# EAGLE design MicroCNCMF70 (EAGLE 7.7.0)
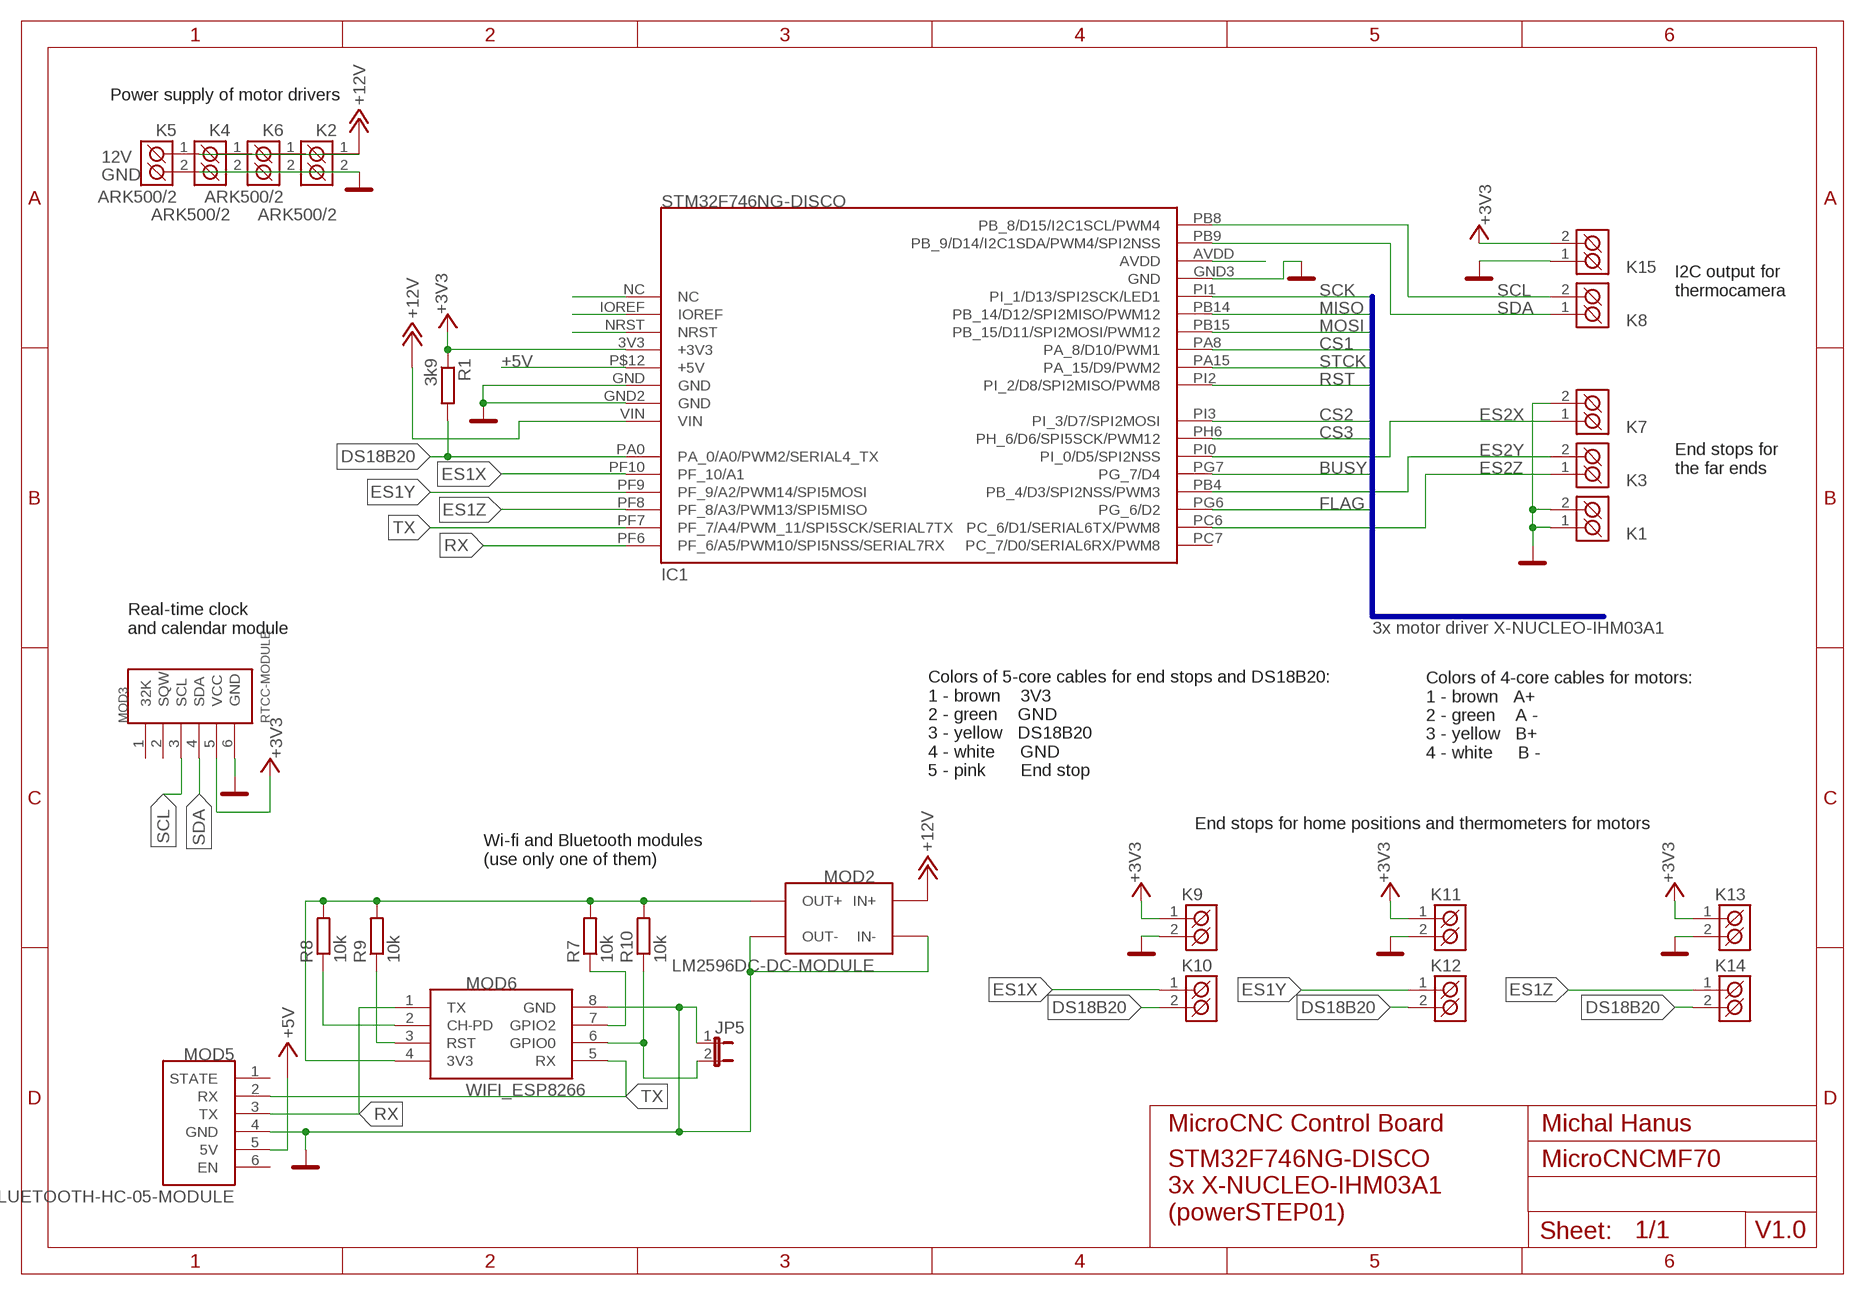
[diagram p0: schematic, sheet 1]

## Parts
IC1  STM32F746NG-DISCO  DISCO+F746NG  [DISCO-F746NG]
JP5  JP1E  [JP1]
K1  ARK500/2  [ARK500/2]
K2  ARK500/2  [ARK500/2]
K3  ARK500/2  [ARK500/2]
K4  ARK500/2  [ARK500/2]
K5  ARK500/2  [ARK500/2]
K6  ARK500/2  [ARK500/2]
K7  ARK500/2  [ARK500/2]
K8  ARK500/2  [ARK500/2]
K9  ARK500/2  [ARK500/2]
K10  ARK500/2  [ARK500/2]
K11  ARK500/2  [ARK500/2]
K12  ARK500/2  [ARK500/2]
K13  ARK500/2  [ARK500/2]
K14  ARK500/2  [ARK500/2]
K15  ARK500/2  [ARK500/2]
MOD2  LM2596DC-DC-MODULE  LM2596DC-DC-MODUL  [LM2596DC-DC-MODUL]
MOD3  RTCC-MODULE  RTCC-MODUL  [RTCC-MODUL]
MOD5  BLUETOOTH-HC-05-MODULE  BLUETOOTH-HC-05  [BLUETOOTH-HC-05]
MOD6  WIFI_ESP8266  [WIFI-ESP8266]
R1  3k9  R  [R0805]
R7  10k  R  [R0805]
R8  10k  R  [R0805]
R9  10k  R  [R0805]
R10  10k  R  [R0805]

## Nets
+3V3: IC1.3V3(+3V3) K9.1(K1) K11.1(K1) K13.1(K1) K15.2(K2) MOD3.5(VCC) R1.1
+5V: IC1.P$12(+5V) MOD5.5(5V)
+12V: IC1.VIN K2.1(K1) K4.1(K1) K5.1(K1) K6.1(K1) MOD2.IN+
BUSY: IC1.PG7(PG_7/D4)
CS1: IC1.PA8(PA_8/D10/PWM1)
CS2: IC1.PI3(PI_3/D7/SPI2MOSI)
CS3: IC1.PH6(PH_6/D6/SPI5SCK/PWM12)
DS18B20: IC1.PA0(PA_0/A0/PWM2/SERIAL4_TX) K10.2(K2) K12.2(K2) K14.2(K2) R1.2
ES1X: IC1.PF10(PF_10/A1) K10.1(K1)
ES1Y: IC1.PF9(PF_9/A2/PWM14/SPI5MOSI) K12.1(K1)
ES1Z: IC1.PF8(PF_8/A3/PWM13/SPI5MISO) K14.1(K1)
ES2X: IC1.PI0(PI_0/D5/SPI2NSS) K7.1(K1)
ES2Y: IC1.PB4(PB_4/D3/SPI2NSS/PWM3) K3.2(K2)
ES2Z: IC1.PC6(PC_6/D1/SERIAL6TX/PWM8) K3.1(K1)
FLAG: IC1.PG6(PG_6/D2)
GND: IC1.GND IC1.GND2(GND) IC1.GND3(GND) JP5.1 K1.1(K1) K1.2(K2) K2.2(K2) K4.2(K2) K5.2(K2) K6.2(K2) K7.2(K2) K9.2(K2) K11.2(K2) K13.2(K2) K15.1(K1) MOD2.IN- MOD2.OUT- MOD3.6(GND) MOD5.4(GND) MOD6.8(GND)
MISO: IC1.PB14(PB_14/D12/SPI2MISO/PWM12)
MOSI: IC1.PB15(PB_15/D11/SPI2MOSI/PWM12)
N$2: IC1.NC
N$3: MOD2.OUT+ MOD6.4(3V3) R7.2 R8.2 R9.2 R10.2
N$4: IC1.IOREF
N$6: IC1.NRST
N$8: IC1.AVDD
N$18: MOD6.2(CH-PD) R8.1
N$20: MOD6.3(RST) R9.1
N$33: JP5.2 MOD6.6(GPIO0) R10.1
N$35: MOD6.7(GPIO2) R7.1
RST: IC1.PI2(PI_2/D8/SPI2MISO/PWM8)
RX: IC1.PF6(PF_6/A5/PWM10/SPI5NSS/SERIAL7RX) MOD5.3(TX) MOD6.1(TX)
SCK: IC1.PI1(PI_1/D13/SPI2SCK/LED1)
SCL: IC1.PB8(PB_8/D15/I2C1SCL/PWM4) K8.2(K2) MOD3.3(SCL)
SDA: IC1.PB9(PB_9/D14/I2C1SDA/PWM4/SPI2NSS) K8.1(K1) MOD3.4(SDA)
STCK: IC1.PA15(PA_15/D9/PWM2)
TX: IC1.PF7(PF_7/A4/PWM_11/SPI5SCK/SERIAL7TX) MOD5.2(RX) MOD6.5(RX)
Unconnected: IC1.PC7(PC_7/D0/SERIAL6RX/PWM8) MOD3.1(32K) MOD3.2(SQW) MOD5.1(STATE) MOD5.6(EN)

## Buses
B$1

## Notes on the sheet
- Power supply of motor drivers
- 12V
- GND
- I2C output for 
  thermocamera
- End stops for 
  the far ends
- Real-time clock 
  and calendar module
- 3x motor driver X-NUCLEO-IHM03A1
- Colors of 4-core cables for motors:
  1 - brown   A+
  2 - green    A -
  3 - yellow   B+
  4 - white     B -
- Colors of 5-core cables for end stops and DS18B20:
  1 - brown    3V3
  2 - green    GND
  3 - yellow   DS18B20
  4 - white     GND
  5 - pink       End stop
- End stops for home positions and thermometers for motors
- Wi-fi and Bluetooth modules
  (use only one of them)
- MicroCNC Control Board | Michal Hanus
- STM32F746NG-DISCO
  3x X-NUCLEO-IHM03A1
  (powerSTEP01)
- V1.0

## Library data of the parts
IC1 = #hahahalib:DISCO+F746NG
JP5 = jumper:JP1E: JUMPER
K1-K15 = #PaJa_konektory:ARK500/2: Svorkovnice - roztec 5mm - dvojita
MOD2 = #hahahalib:LM2596DC-DC-MODUL
MOD3 = #hahahalib:RTCC-MODUL
MOD5 = #hahahalib:BLUETOOTH-HC-05
MOD6 = #hahahalib:WIFI_ESP8266
R1 R7-R10 = eagle-ltspice:R: RESISTOR, European symbol; SPICEMODEL: NONE; SPICEPREFIX: R

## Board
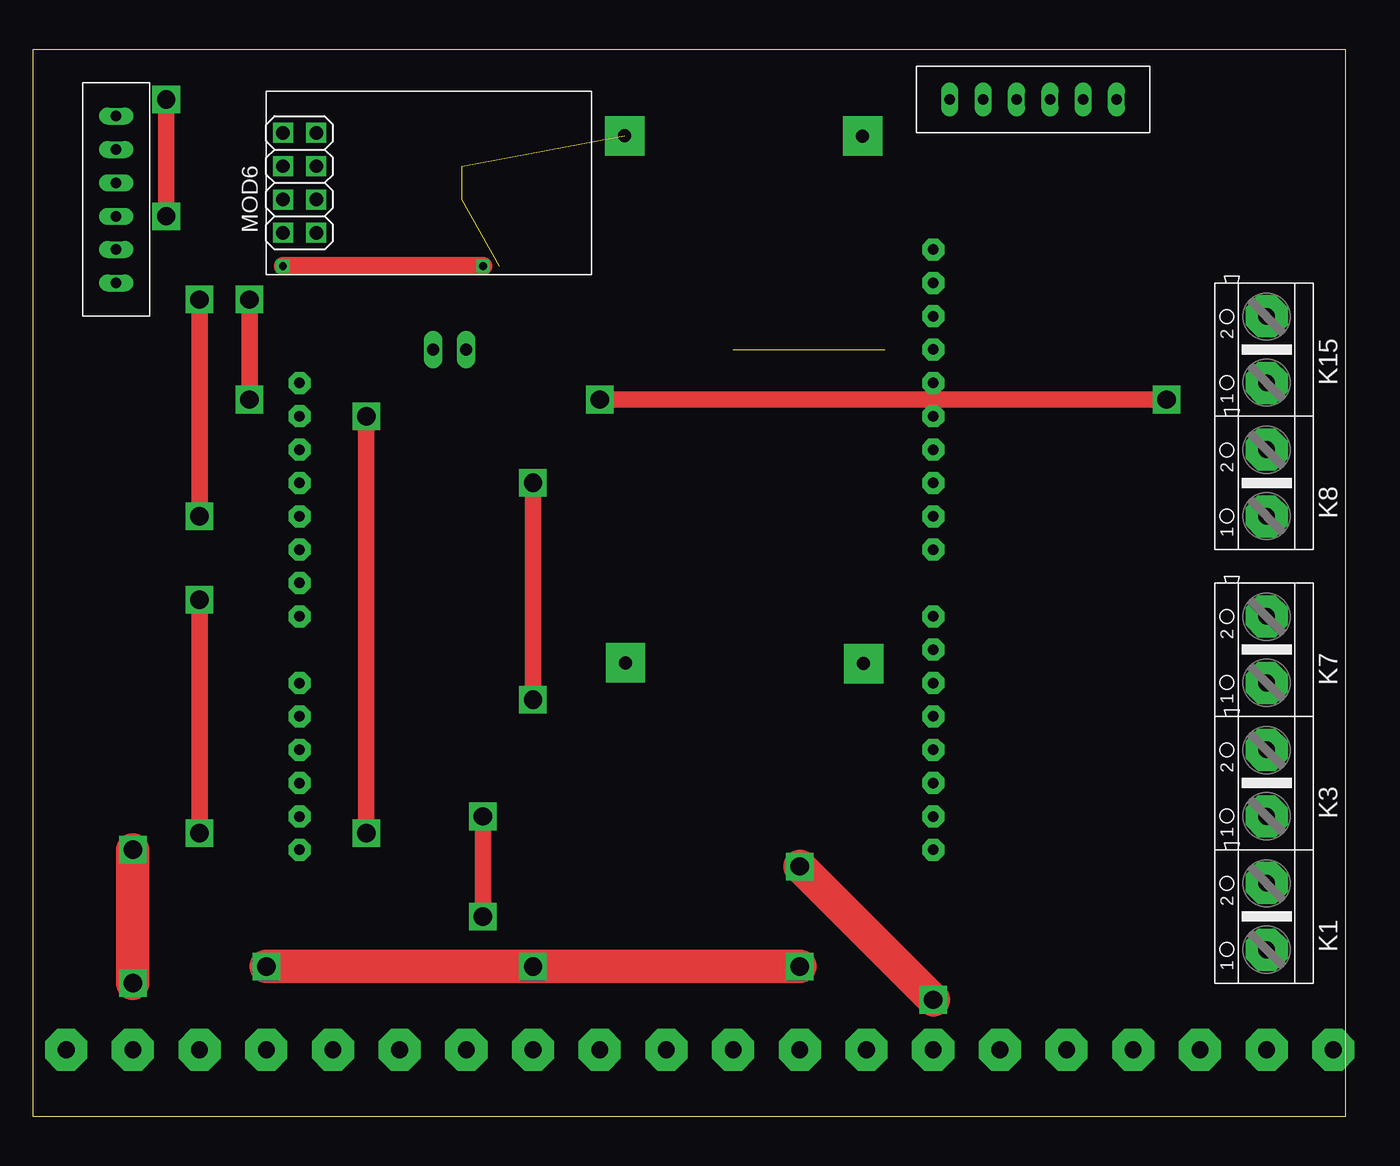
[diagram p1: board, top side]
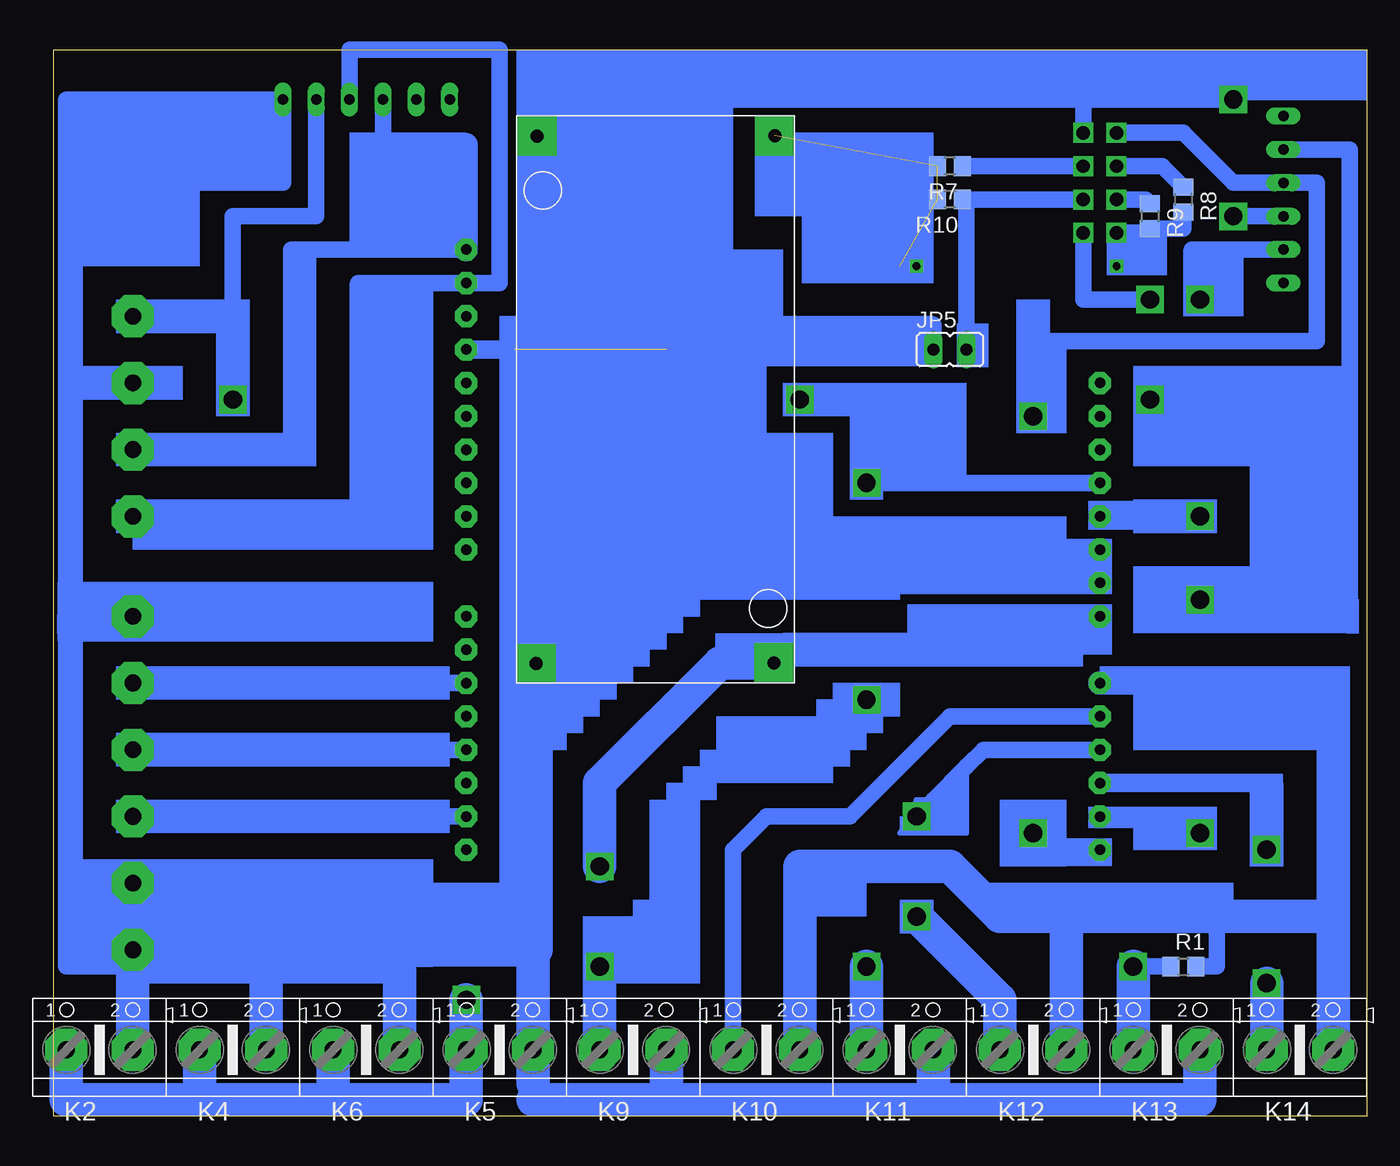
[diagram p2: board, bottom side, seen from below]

Size 100 x 81.27 mm. Coordinates in mm from the lower left corner, seen from the top.
Outline: 0,0 100,0 100,81.27 0,81.27 0,0
Copper layers (1*16): Top 0.035mm / dielectric 1.5mm / Bottom 0.035mm
Design rules "default *": minimum track width 10mil, minimum drill 24mil, track to track 1mm, track to pad 1mm, pad to pad 1mm, via to via 1mm, smd to smd 1mm, copper to edge 40mil, drill to drill 8mil, minimum pad ring 10mil, minimum via ring 8mil, stop-mask expansion 4mil, vias tented up to drill 0mil, thermal gap 10mil

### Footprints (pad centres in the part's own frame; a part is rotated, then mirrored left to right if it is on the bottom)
DISCO-F746NG = drill 0.8 pad 1.676 octagon: 3V3 0,33.02; AVDD 48.26,45.72; GND 0,27.94; GND2 0,25.4; GND3 48.26,43.18; IOREF 0,38.1; NC 0,40.64; NRST 0,35.56; P$12 0,30.48; PA0 0,17.78; PA8 48.26,33.02; PA15 48.26,30.48; PB4 48.26,12.7; PB8 48.26,50.8; PB9 48.26,48.26; PB14 48.26,38.1; PB15 48.26,35.56; PC6 48.26,7.62; PC7 48.26,5.08; PF6 0,5.08; PF7 0,7.62; PF8 0,10.16; PF9 0,12.7; PF10 0,15.24; PG6 48.26,10.16; PG7 48.26,15.24; PH6 48.26,20.32; PI0 48.26,17.78; PI1 48.26,40.64; PI2 48.26,27.94; PI3 48.26,22.86; VIN 0,22.86
JP1 = drill 0.914 long: 1 0,-1.27; 2 0,1.27
ARK500/2 = drill 1.27 pad 3.2 octagon: 1 -2.54,0; 2 2.54,0
LM2596DC-DC-MODUL = drill 1 pad 3 square: IN+ 1.54,19.62; IN- 1.48,1.49; OUT+ 41.68,19.69; OUT- 41.66,1.57
RTCC-MODUL = drill 0.8 pad 1.016 long: 1 -5.08,7.62; 2 -5.08,5.08; 3 -5.08,2.54; 4 -5.08,0; 5 -5.08,-2.54; 6 -5.08,-5.08
BLUETOOTH-HC-05 = drill 0.8 pad 1.016 long: 1 0,5.08; 2 0,2.54; 3 0,0; 4 0,-2.54; 5 0,-5.08; 6 0,-7.62
WIFI-ESP8266 = drill 1.016 square: 1 -3.81,3.81; 2 -3.81,1.27; 3 -3.81,-1.27; 4 -3.81,-3.81; 5 -1.27,-3.81; 6 -1.27,-1.27; 7 -1.27,1.27; 8 -1.27,3.81
R0805 = smd 1.3 x 1.5: 1 -0.95,0; 2 0.95,0

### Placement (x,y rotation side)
IC1  20.32,15.24 0 top
JP5  31.75,58.42 270 bottom
K1  93.98,15.24 90 top
K2  96.52,5.08 0 bottom
K3  93.98,25.4 90 top
K4  86.36,5.08 0 bottom
K5  66.04,5.08 0 bottom
K6  76.2,5.08 0 bottom
K7  93.98,35.56 90 top
K8  93.98,48.26 90 top
K9  55.88,5.08 0 bottom
K10  45.72,5.08 0 bottom
K11  35.56,5.08 0 bottom
K12  25.4,5.08 0 bottom
K13  15.24,5.08 0 bottom
K14  5.08,5.08 0 bottom
K15  93.98,58.42 90 top
MOD2  64.77,33.02 90 top
MOD3  77.47,82.55 90 top
MOD5  6.35,71.12 0 top
MOD6  22.86,71.12 0 top
R1  13.97,11.43 0 bottom
R7  31.75,72.39 180 bottom
R8  13.97,69.85 270 bottom
R9  16.51,68.58 270 bottom
R10  31.75,69.85 180 bottom

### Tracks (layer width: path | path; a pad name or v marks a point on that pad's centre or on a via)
+3V3  (via drill 1.4)
  Top 1.27: v43.18,54.61 v86.36,54.61 | v38.1,31.75 v38.1,48.26
  Top 2.54: v17.78,11.43 v38.1,11.43 v58.42,11.43 v17.78,11.43
  Bottom 1.27: MOD3.5 80.01,68.58 86.36,68.58 86.36,60.96 | IC1.3V3 31.75,48.26 | 31.75,48.26 31.75,54.61 v43.18,54.61 | 58.42,12.7 52.07,12.7 52.07,24.13 49.53,26.67 41.91,26.67 v38.1,31.75 | v38.1,48.26 31.75,48.26 | R1.1 v17.78,11.43 | v86.36,54.61 86.36,60.96 | 86.36,60.96 K15.2
  Bottom 2.54: K13.1 v17.78,11.43 | v38.1,11.43 K11.1 | K9.1 v58.42,11.43 58.42,12.7
+5V  (via drill 1.4)
  Top 1.27: v12.7,62.23 v12.7,45.72
  Bottom 1.27: MOD5.5 12.7,66.04 | 12.7,66.04 v12.7,62.23 | v12.7,45.72 IC1.P$12 | 12.7,66.04 13.34,66.04
+12V  (via drill 1.4)
  Top 2.54: v68.58,8.89 v58.42,19.05
  Bottom 1.27: MOD2.IN+ 45.72,35.56 45.72,35.83 33.02,35.83 33.02,38.1 IC1.VIN
  Bottom 2.54: K4.1 88.9,1.27 | 88.9,1.27 78.74,1.27 | 78.74,1.27 K6.1 | K2.1 99.06,1.27 88.9,1.27 | 78.74,1.27 68.58,1.27 K5.1 v68.58,8.89 | 45.15,34.29 MOD2.IN+ 49.26,34.56 58.42,25.4 v58.42,19.05
DS18B20
  Bottom 1.27: 2.54,15.24 2.54,33.02 | R1.2 11.43,11.43 11.43,15.24
  Bottom 1.778: 2.54,33.02 IC1.PA0
  Bottom 2.54: K14.2 2.54,15.24 11.43,15.24 22.86,15.24 | K12.2 22.86,15.24 | 22.86,15.24 27.94,15.24 31.75,19.05 43.18,19.05 K10.2
ES1X
  Bottom 1.27: K10.1 48.26,20.32 45.72,22.86 39.37,22.86 31.75,30.48 IC1.PF10
ES1Y  (via drill 1.4)
  Top 1.27: v34.29,15.24 v34.29,22.86
  Bottom 0.406: 30.48,26.67 33.02,22.86 30.48,25.4 | 30.48,25.4 30.48,26.67 | 30.48,25.4 30.48,21.59 35.56,21.59 34.29,24.13 33.02,24.13 | 30.48,26.67 31.75,22.86
  Bottom 1.27: v34.29,22.86 33.02,24.13 30.48,26.67 29.21,27.94 IC1.PF9
  Bottom 2.54: K12.1 27.94,8.89 v34.29,15.24
ES1Z  (via drill 1.4)
  Top 2.54: v7.62,10.16 v7.62,20.32
  Bottom 1.422: v7.62,20.32 7.62,25.4 IC1.PF8
  Bottom 2.54: K14.1 v7.62,10.16
ES2X
  Bottom 1.27: K7.1 IC1.PI0
ES2Y
  Bottom 1.27: IC1.PB4 K3.2
ES2Z
  Bottom 1.27: IC1.PC6 K3.1
GND  (via drill 1.4)  (1 unrouted)
  Top 1.27: v10.16,68.58 v10.16,77.47
  Bottom 1.27: 63.5,2.54 63.5,1.27 | 53.34,43.18 53.34,58.42 | 53.34,74.68 53.34,58.42 | 53.34,58.42 JP5.1 33.02,60.33 | MOD2.OUT- 62.23,74.68 | 62.23,74.68 53.34,74.68 | IC1.GND2 IC1.GND 53.34,43.18 | MOD5.4 v10.16,68.58 | v10.16,77.47 21.59,77.47 | MOD6.8 21.59,77.47 | 21.59,77.47 53.34,77.47 53.34,74.68 | MOD2.IN- 63.28,43.18 53.34,43.18 | 62.23,71.12 62.23,74.68 | K1.1 K1.2 | 99.06,71.12 82.55,71.12 MOD3.6 99.06,77.47 99.06,71.12 | 99.06,55.88 99.06,36.9 99.06,11.43 93.98,11.43 | 99.06,55.88 K15.1 | 99.06,55.88 99.06,71.12
  Bottom 1.422: IC1.GND3 64.9,58.42 64.9,58.2 | K7.2 99.06,38.1 99.06,36.9
  Bottom 2.54: 63.5,1.27 53.34,1.27 | 53.34,1.27 K9.2 | K13.2 12.7,1.27 33.02,1.27 | K11.2 33.02,1.27 | 33.02,1.27 53.34,1.27 | 73.66,12.7 63.5,12.7 | 73.66,12.7 83.82,11.43 | 63.5,12.7 K5.2 63.5,2.54 | 73.66,12.7 K6.2 | 83.82,11.43 K4.2 | 93.98,11.43 K2.2 | 93.98,11.43 83.82,11.43 | MOD2.IN- 63.28,12.7 63.5,12.7 | 93.98,11.43 K1.1
N$3  (via drill 0.6)  (3 unrouted)
  Top 1.422: v19.05,64.77 v34.29,64.77
  Bottom 1.27: 45.08,74.61 MOD2.OUT+ | R8.2 13.97,67.63 R9.2 arc90 16.83,67.31 MOD6.4
  Bottom 1.422: MOD6.4 v19.05,64.77 | v34.29,64.77 35.56,64.77
N$18
  Bottom 1.27: R8.1 15.56,72.39 MOD6.2
N$20
  Bottom 1.27: R9.1 16.83,69.85 MOD6.3
N$33
  Bottom 1.27: MOD6.6 R10.1 30.48,69.53 JP5.2
N$35
  Bottom 1.27: MOD6.7 R7.1
RX  (via drill 1.4)
  Top 1.27: v25.4,21.59 v25.4,53.34
  Bottom 1.27: IC1.PF6 25.4,20.32 v25.4,21.59 | v25.4,53.34 25.4,59.05 3.81,59.05 3.81,71.12 MOD5.3 10.16,71.12 13.97,74.93 MOD6.1 17.78,74.93
SCL
  Bottom 1.27: IC1.PB8 74.93,66.04 | 74.93,66.04 80.01,66.04 81.28,66.04 | 81.28,66.04 81.28,50.8 K8.2 | MOD3.3 74.93,66.04 | 81.28,66.04 81.92,66.04
  Bottom 1.778: IC1.PB8 68.58,74.04
SDA
  Bottom 1.27: 76.2,63.5 76.2,45.72 K8.1 | 76.2,63.5 IC1.PB9 66.04,63.5 66.04,81.28 77.47,81.28 MOD3.4 | 76.2,63.5 76.83,63.5
TX  (via drill 1.4)
  Top 1.27: v12.7,21.59 v12.7,39.37 | v16.51,62.23 v16.51,54.61
  Bottom 1.27: IC1.PF7 12.7,22.86 v12.7,21.59 | v12.7,39.37 1.27,39.37 1.27,55.88 | 1.27,55.88 1.27,73.66 MOD5.2 | MOD6.5 21.59,62.23 v16.51,62.23 | v16.51,54.61 16.51,55.88 1.27,55.88
(copper drawn outside any net)
  shapes: Bottom area x143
